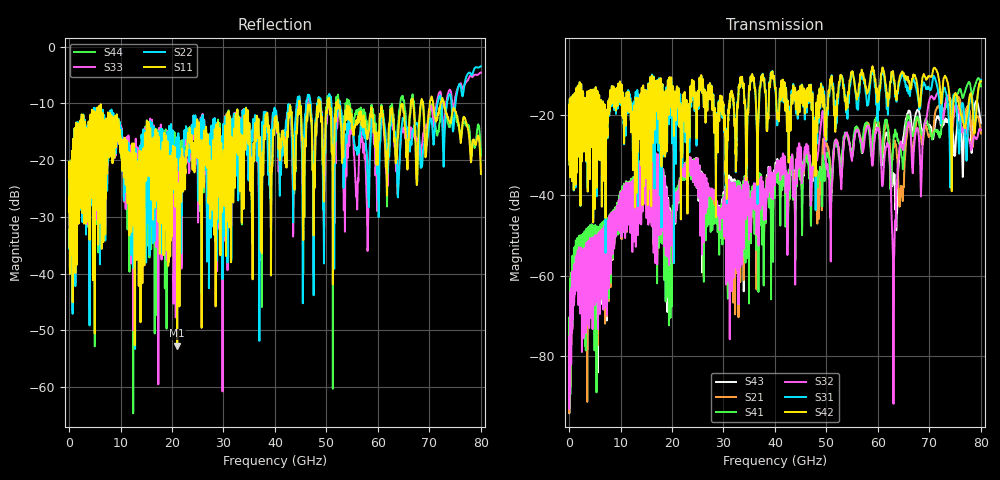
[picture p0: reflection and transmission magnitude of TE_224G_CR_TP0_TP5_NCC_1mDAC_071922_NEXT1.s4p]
!! Reference: tracy_3df_01a_2207
!! CHANNEL DESCRIPTION: TP0_TP5 CR Channel using 1meter DAC, CABLED NCC Host
!! MODEL DESCRIPTION: s4p, NEXT1
!! CONNECTOR DESCRIPTION: OSFP 200G OTB, NCC Socket
!! CABLE DESCRIPTION: 1meter 26AWG Cable
!! MODEL STATUS: Developmental
!! PORT DEFINITIONS:
!! Port  1  ----->  Side A  Side B  <-----  Port  2
!! Port  3  ----->  Side A  Side B  <-----  Port  4
# GHz S MA R 50
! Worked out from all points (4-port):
!   8000 points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, 10 MHz to 80 GHz, reference 50 ohm
!   strongest paths, dB at 10 MHz, 20.01 GHz, 40.01 GHz, 60.01 GHz, 80 GHz:
!     S42: -24.5, -20.2, -13.4, -14.6, -11.7
!     S31: -24.5, -26.1, -13.7, -17.6, -11.4
!     S32: -80.4, -50.3, -35.9, -23.4, -23.8
!     S41: -77.9, -50.9, -36.9, -22.5, -13.0
!     S21: -79.4, -49.4, -35.8, -21.6, -24.7
!     S43: -79.5, -54.5, -35.3, -22.8, -22.1
!   lowest |S11| = -52.7 dB at 21.01 GHz (marker M1), VSWR 1.00, Z = 50 + j0.231 ohm
!   |S11| at or under -10 dB: start of sweep to 44.68 GHz; 52.32 GHz to 66.38 GHz (14.06 GHz wide, 23.7 % of centre); 72.83 GHz to end of sweep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
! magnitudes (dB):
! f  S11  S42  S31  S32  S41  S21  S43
! 10 MHz  -23.1  -24.5  -24.5  -80.4  -77.9  -79.4  -79.5
! 14.55 GHz  -22.6  -23.4  -28.6  -29.3  -29.4  -29.4  -29.2
! 21.01 GHz  -52.7  -15.1  -17.3  -41.6  -41.7  -40.9  -41.9
! 58.05 GHz  -15.6  -14.3  -17.5  -22.8  -22.6  -22.1  -22.9
! 63.07 GHz  -13.5  -11.3  -12.0  -60.1  -25.2  -28.2  -36.9
! 65.88 GHz  -16.5  -11.2  -13.9  -22.0  -20.6  -23.2  -19.4
! 80 GHz  -22.4  -11.7  -11.4  -23.8  -13.0  -24.7  -22.1
